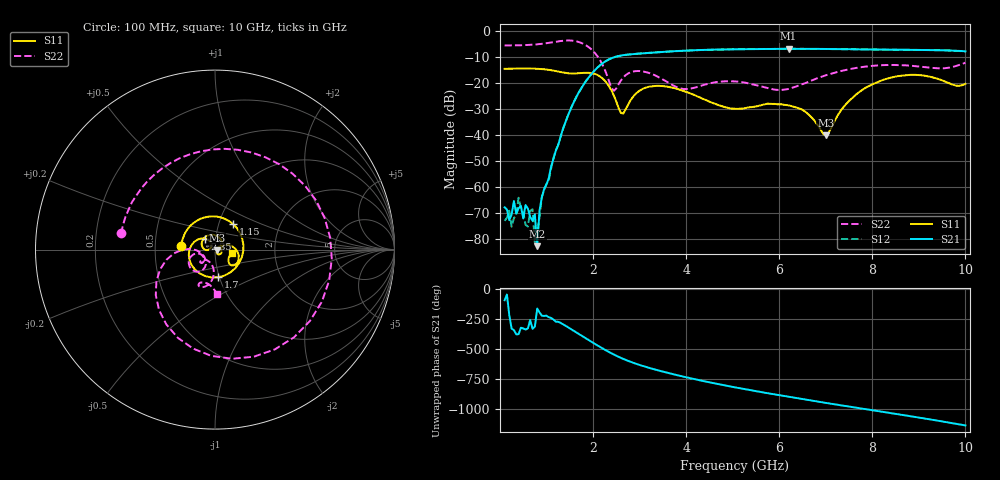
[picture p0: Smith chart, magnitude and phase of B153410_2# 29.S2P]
!  2-Port S-parameters saved by WinCal
! VAR MeasName=S-Parameters (CALIBRATED_DATA) read from VNA (N5245A)
! VAR MeasDate=2016-12-23 10:00:50
! VAR NAME=B153410_2# 29
! VAR FILENAME=B153410_2# 29.S2P
! VAR DATE=2016-12-23 10:00:50
! VAR PHYS_PORTS=1,2
# Hz S DB R 50
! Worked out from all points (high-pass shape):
!   199 points, 100 MHz to 10 GHz, reference 50 ohm
!   highest |S21| = -6.79 dB at 6.2 GHz (marker M1); lowest = -82.8 dB at 800 MHz (marker M2)
!   |S21| within 3 dB of the highest: 2.5 GHz to end of sweep
!   lowest |S11| = -40.1 dB at 7 GHz (marker M3), VSWR 1.02, Z = 50.9 - j0.341 ohm
!   |S11| at or under -10 dB: start of sweep to end of sweep
!   |S22| runs from -23.0 to -3.6 dB; largest |S21 - S12| = 0.0035
!   S11 on the Smith chart (normalised r, x): 100 MHz: 0.68, +0.03; 1.15 GHz: 1.17, +0.34; 1.7 GHz: 0.98, -0.31; 2.35 GHz: 0.88, +0.11; 10 GHz: 1.21, -0.05
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1e8  -14.51 173.1  -67.86 -91.5  -73.07 50.8  -5.51 170.2
2.5e8  -14.45 161.8  -70.72 31.0  -75.33 -8.0  -5.51 155.4
4e8  -14.40 149.7  -68.22 -15.8  -64.17 97.3  -5.45 139.8
5.5e8  -14.38 136.2  -66.98 22.8  -74.59 -105.2  -5.36 123.1
7e8  -14.43 121.1  -73.05 29.7  -68.61 73.5  -5.21 104.8
7.5e8  -14.44 115.3  -70.56 47.6  -81.56 71.9  -5.14 98.3
8e8  -14.50 109.3  -82.82 -160.6  -77.07 150.2  -5.06 91.5
9e8  -14.60 96.0  -63.99 138.8  -63.84 165.8  -4.88 77.1
1.15e9  -15.19 54.2  -49.17 106.5  -48.84 107.3  -4.22 35.2
1.4e9  -16.06 -3.3  -35.40 57.1  -35.40 57.5  -3.62 -15.1
1.7e9  -16.18 -84.2  -23.41 -16.1  -23.44 -15.8  -4.21 -81.0
1.75e9  -16.11 -97.2  -21.93 -28.2  -21.88 -28.1  -4.54 -91.9
2e9  -16.28 -157.6  -15.80 -87.8  -15.79 -87.7  -7.62 -142.5
2.35e9  -21.45 133.6  -10.79 -166.1  -10.79 -166.0  -19.60 -178.4
2.65e9  -31.72 163.9  -9.24 137.6  -9.25 137.6  -17.83 -120.7
3.4e9  -21.05 126.0  -8.12 41.8  -8.12 41.8  -17.64 -165.8
5.05e9  -29.90 0.2  -6.97 -99.9  -6.98 -99.7  -19.36 -140.1
6.2e9  -28.59 -45.6  -6.79 -178.7  -6.81 -178.6  -22.26 -111.0
6.7e9  -33.29 -61.4  -6.81 149.2  -6.83 149.2  -18.96 -93.9
7e9  -40.13 -19.8  -6.85 130.2  -6.87 130.3  -16.99 -93.1
8.35e9  -18.14 -4.7  -7.14 47.7  -7.13 48.0  -13.00 -110.7
1e10  -20.29 -12.4  -7.77 -58.3  -7.80 -58.1  -12.14 -87.7
